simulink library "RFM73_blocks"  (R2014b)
settings: Solver=ode45  StartTime=0.0  StopTime=10.0  RelTol=1e-3
undefined symbols (not defined in the file): B, bin2dec, Model
libraries: simulink x5, RFM73_blocks x1, commutil2 x1, embdlinuxlib x1

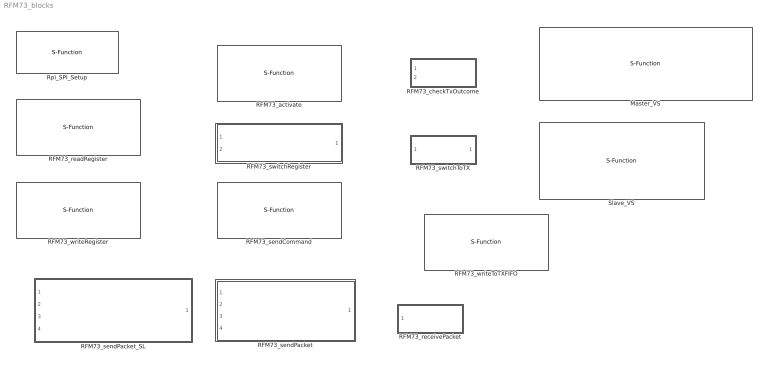
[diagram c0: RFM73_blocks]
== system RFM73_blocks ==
  Master_VS : S-Function  InitFcn=try, set_param(gcb,'FunctionName','RFM73_Master_VS'), end  FunctionName=RFM73_Master_VS  SFunctionModules=RFM73_Master_VS_wrapper  EnableBusSupport=off
  RFM73_activate : S-Function  InitFcn=try, set_param(gcb,'FunctionName','activate'), end  FunctionName=activate  SFunctionModules=activate_wrapper  EnableBusSupport=off
  RFM73_checkTxOutcome : Subsystem  TreatAsAtomicUnit=on
  RFM73_readRegister : S-Function  InitFcn=try, set_param(gcb,'FunctionName','readRegister'), end  FunctionName=readRegister  SFunctionModules=readRegister_wrapper  EnableBusSupport=off
  RFM73_receivePacket : Subsystem  TreatAsAtomicUnit=on
  RFM73_sendCommand : S-Function  InitFcn=try, set_param(gcb,'FunctionName','sendCommand'), end  FunctionName=sendCommand  SFunctionModules=sendCommand_wrapper  EnableBusSupport=off
  RFM73_sendPacket : Subsystem  TreatAsAtomicUnit=on
  RFM73_sendPacket_SL : Subsystem  TreatAsAtomicUnit=on
  RFM73_switchRegister : Subsystem
  RFM73_switchToTX : Subsystem  TreatAsAtomicUnit=on
  RFM73_writeRegister : S-Function  InitFcn=try, set_param(gcb,'FunctionName','writeRegister'), end  FunctionName=writeRegister  SFunctionModules=writeRegister_wrapper  EnableBusSupport=off
  RFM73_writeToTXFIFO : S-Function  InitFcn=try, set_param(gcb,'FunctionName','writeToTXFIFO'), end  FunctionName=writeToTXFIFO  SFunctionModules=writeToTXFIFO_wrapper  EnableBusSupport=off
  Rpi_SPI_Setup : S-Function  InitFcn=try, set_param(gcb,'FunctionName','SPI_interface_setup'), end  FunctionName=SPI_interface_setup  SFunctionModules=SPI_interface_setup_wrapper  EnableBusSupport=off
  Slave_VS : S-Function  InitFcn=try, set_param(gcb,'FunctionName','RFM73_Slave_VS'), end  FunctionName=RFM73_Slave_VS  SFunctionModules=RFM73_Slave_VS_wrapper  EnableBusSupport=off

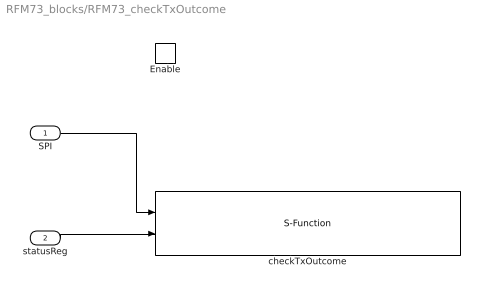
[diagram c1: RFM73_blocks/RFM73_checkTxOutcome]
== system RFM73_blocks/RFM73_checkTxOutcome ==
  SPI : Inport
  statusReg : Inport  Port=2
  Enable : EnablePort
  checkTxOutcome : S-Function  InitFcn=try, set_param(gcb,'FunctionName','checkTxOutcome'), end  FunctionName=checkTxOutcome  SFunctionModules=checkTxOutcome_wrapper  EnableBusSupport=off
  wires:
  SPI/1 -> checkTxOutcome/1
  statusReg/1 -> checkTxOutcome/2

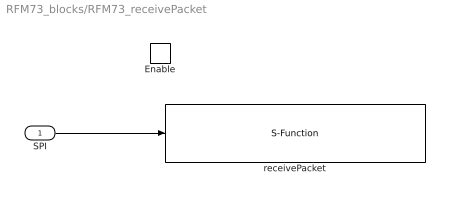
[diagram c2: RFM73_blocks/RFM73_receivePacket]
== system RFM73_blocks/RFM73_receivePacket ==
  SPI : Inport
  Enable : EnablePort
  receivePacket : S-Function  InitFcn=try, set_param(gcb,'FunctionName','receivePacket'), end  FunctionName=receivePacket  SFunctionModules=receivePacket_wrapper  EnableBusSupport=off
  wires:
  SPI/1 -> receivePacket/1

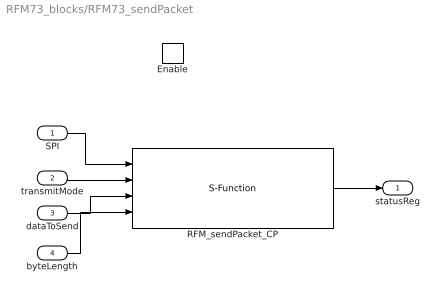
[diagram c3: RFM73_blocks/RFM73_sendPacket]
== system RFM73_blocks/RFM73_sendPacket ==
  SPI : Inport
  transmitMode : Inport  Port=2
  dataToSend : Inport  Port=3
  byteLength : Inport  Port=4
  Enable : EnablePort
  RFM_sendPacket_CP : S-Function  InitFcn=try, set_param(gcb,'FunctionName','sendPacket_CP'), end  FunctionName=sendPacket_CP  SFunctionModules=sendPacket_CP_wrapper  EnableBusSupport=off
  statusReg : Outport
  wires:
  RFM_sendPacket_CP/1 -> statusReg/1
  SPI/1 -> RFM_sendPacket_CP/1
  transmitMode/1 -> RFM_sendPacket_CP/2
  dataToSend/1 -> RFM_sendPacket_CP/3
  byteLength/1 -> RFM_sendPacket_CP/4

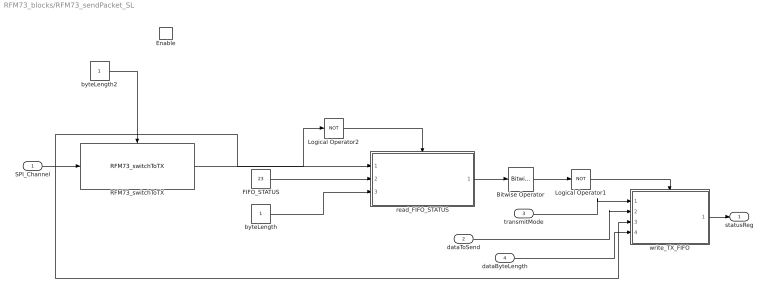
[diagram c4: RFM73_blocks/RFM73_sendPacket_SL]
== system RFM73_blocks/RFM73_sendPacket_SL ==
  SPI_Channel : Inport
  dataToSend : Inport  Port=2  OutDataTypeStr=uint8
  transmitMode : Inport  Port=3
  dataByteLength : Inport  Port=4  OutDataTypeStr=uint8
  Enable : EnablePort
  Bitwise Operator : simulink/Logic and Bit Operations/Bitwise Operator  logicop=AND  UseBitMask=on  BitMask=bin2dec('00000010')  BitMaskRealWorld=Stored Integer
  FIFO_STATUS : Constant  Value=23
  Logical Operator1 : Logic  Operator=NOT  AllPortsSameDT=off  OutDataTypeStr=boolean
  Logical Operator2 : Logic  Operator=NOT  AllPortsSameDT=off  OutDataTypeStr=boolean
  RFM73_switchToTX : RFM73_blocks/RFM73_switchToTX
      link override RFM73_sendCommand: FunctionName=sendCommand  SFunctionModules=sendCommand_wrapper
      link override RFM73_writeConfigRegister: FunctionName=writeRegister  SFunctionModules=writeRegister_wrapper
  byteLength : Constant
  byteLength2 : Constant
  read_FIFO_STATUS : Subsystem  TreatAsAtomicUnit=on
  write_TX_FIFO : Subsystem  TreatAsAtomicUnit=on
  statusReg : Outport
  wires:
  write_TX_FIFO/1(statusReg) -> statusReg/1
  dataByteLength/1 -> write_TX_FIFO/4(byteLength)
  transmitMode/1 -> write_TX_FIFO/1(type)
  dataToSend/1 -> write_TX_FIFO/2(data)
  Logical Operator1/1 -> write_TX_FIFO/Enable
  Bitwise Operator/1 -> Logical Operator1/1
  read_FIFO_STATUS/1(regContent) -> Bitwise Operator/1
  Logical Operator2/1 -> read_FIFO_STATUS/Enable
  RFM73_switchToTX/1 -> Logical Operator2/1
  byteLength/1 -> read_FIFO_STATUS/3(byteLength)
  FIFO_STATUS/1 -> read_FIFO_STATUS/2(regAddress)
  SPI_Channel/1 -> RFM73_switchToTX/1, read_FIFO_STATUS/1(SPI_Channel), write_TX_FIFO/3(SPI_Channel)
  byteLength2/1 -> RFM73_switchToTX/Enable

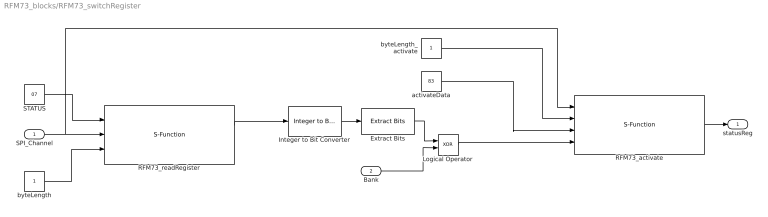
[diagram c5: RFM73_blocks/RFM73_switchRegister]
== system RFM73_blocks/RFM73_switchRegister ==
  SPI_Channel : Inport
  Bank : Inport  Port=2
  Extract Bits : simulink/Logic and Bit Operations/Extract Bits  bitsToExtract=Range of bits  numBits=8  bitIdxRange=[7]  outScalingMode=Preserve fixed-point scaling
  Integer to Bit Converter : commutil2/Integer to Bit Converter  nbits=8  signedInputValues=Unsigned  bitOrder=MSB first  outDtype=Inherit via internal rule
  Logical Operator : Logic  Operator=XOR  IconShape=distinctive  AllPortsSameDT=off  OutDataTypeStr=boolean
  RFM73_activate : S-Function  InitFcn=try, set_param(gcb,'FunctionName','activate'), end  FunctionName=activate  SFunctionModules=activate_wrapper  EnableBusSupport=off
  RFM73_readRegister : S-Function  InitFcn=try, set_param(gcb,'FunctionName','readRegister'), end  FunctionName=readRegister  SFunctionModules=readRegister_wrapper  EnableBusSupport=off
  STATUS : Constant  Value=07
  activateData : Constant  Value=83
  byteLength : Constant
  byteLength_activate : Constant
  statusReg : Outport
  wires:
  SPI_Channel/1 -> RFM73_activate/1, RFM73_readRegister/2
  STATUS/1 -> RFM73_readRegister/1
  byteLength/1 -> RFM73_readRegister/3
  RFM73_readRegister/1 -> Integer to Bit Converter/1
  Integer to Bit Converter/1 -> Extract Bits/1
  Extract Bits/1 -> Logical Operator/1
  Bank/1 -> Logical Operator/2
  byteLength_activate/1 -> RFM73_activate/2
  activateData/1 -> RFM73_activate/3
  Logical Operator/1 -> RFM73_activate/4
  RFM73_activate/1 -> statusReg/1

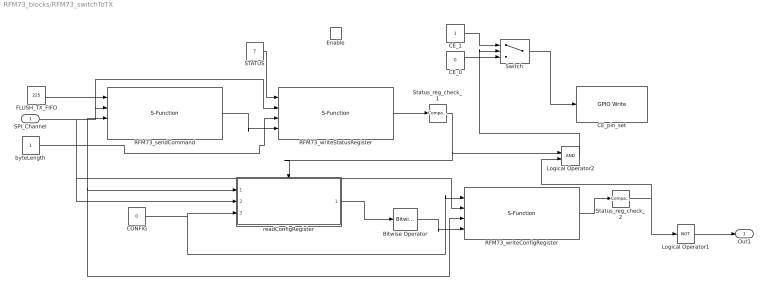
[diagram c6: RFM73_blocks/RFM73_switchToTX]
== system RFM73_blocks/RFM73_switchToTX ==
  SPI_Channel : Inport
  Enable : EnablePort
  Bitwise Operator : simulink/Logic and Bit Operations/Bitwise Operator  logicop=AND  UseBitMask=on  BitMask=bin2dec('11111110')  BitMaskRealWorld=Stored Integer
  CE_0 : Constant  Value=0  OutDataTypeStr=boolean
  CE_1 : Constant  OutDataTypeStr=boolean
  CE_pin_set : embdlinuxlib/GPIO Write  board=Model B+  gpio=23  direction=Output  blockPlatform=Raspberry Pi
  CONFIG : Constant  Value=0
  FLUSH_TX_FIFO : Constant  Value=225
  Logical Operator1 : Logic  Operator=NOT  AllPortsSameDT=off  OutDataTypeStr=boolean
  Logical Operator2 : Logic  AllPortsSameDT=off  OutDataTypeStr=fixdt(0,16)
  RFM73_sendCommand : S-Function  InitFcn=try, set_param(gcb,'FunctionName','sendCommand'), end  FunctionName=sendCommand  SFunctionModules=sendCommand_wrapper  EnableBusSupport=off
  RFM73_writeConfigRegister : S-Function  InitFcn=try, set_param(gcb,'FunctionName','writeRegister'), end  FunctionName=writeRegister  SFunctionModules=writeRegister_wrapper  EnableBusSupport=off
  RFM73_writeStatusRegister : S-Function  InitFcn=try, set_param(gcb,'FunctionName','writeRegister'), end  FunctionName=writeRegister  SFunctionModules=writeRegister_wrapper  EnableBusSupport=off
  STATUS : Constant  Value=7
  Status_reg_check_1 : simulink/Logic and Bit Operations/Compare To Constant  relop===  const=14  OutDataTypeStr=uint8
  Status_reg_check_2 : simulink/Logic and Bit Operations/Compare To Constant  relop===  const=14  OutDataTypeStr=uint8
  Switch : Switch  Criteria=u2 ~= 0
  byteLength : Constant
  readConfigRegister : Subsystem  TreatAsAtomicUnit=on
  Out1 : Outport
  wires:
  SPI_Channel/1 -> RFM73_writeConfigRegister/2, readConfigRegister/2(SPI_Channel), RFM73_writeStatusRegister/2, RFM73_sendCommand/2
  FLUSH_TX_FIFO/1 -> RFM73_sendCommand/1
  byteLength/1 -> RFM73_writeConfigRegister/3, readConfigRegister/1(byteLength), RFM73_writeStatusRegister/3, RFM73_sendCommand/3
  STATUS/1 -> RFM73_writeStatusRegister/1
  RFM73_sendCommand/1 -> RFM73_writeStatusRegister/4
  RFM73_writeStatusRegister/1 -> Status_reg_check_1/1
  Status_reg_check_1/1 -> readConfigRegister/Enable, Logical Operator2/1
  CONFIG/1 -> RFM73_writeConfigRegister/1, readConfigRegister/3(regAddress)
  readConfigRegister/1(regContent) -> Bitwise Operator/1
  Bitwise Operator/1 -> RFM73_writeConfigRegister/4
  RFM73_writeConfigRegister/1 -> Status_reg_check_2/1
  Status_reg_check_2/1 -> Logical Operator2/2, Logical Operator1/1
  Logical Operator1/1 -> Out1/1
  CE_0/1 -> Switch/3
  CE_1/1 -> Switch/1
  Switch/1 -> CE_pin_set/1
  Logical Operator2/1 -> Switch/2

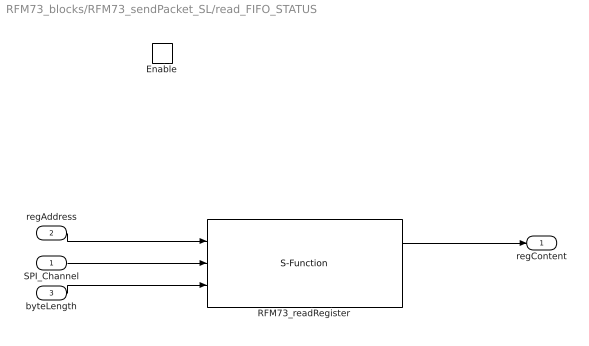
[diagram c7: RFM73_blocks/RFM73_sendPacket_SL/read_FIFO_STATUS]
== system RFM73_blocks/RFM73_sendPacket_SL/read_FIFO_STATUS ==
  SPI_Channel : Inport
  regAddress : Inport  Port=2
  byteLength : Inport  Port=3
  Enable : EnablePort
  RFM73_readRegister : S-Function  InitFcn=try, set_param(gcb,'FunctionName','readRegister'), end  FunctionName=readRegister  SFunctionModules=readRegister_wrapper  EnableBusSupport=off
  regContent : Outport
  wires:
  byteLength/1 -> RFM73_readRegister/3
  regAddress/1 -> RFM73_readRegister/1
  SPI_Channel/1 -> RFM73_readRegister/2
  RFM73_readRegister/1 -> regContent/1

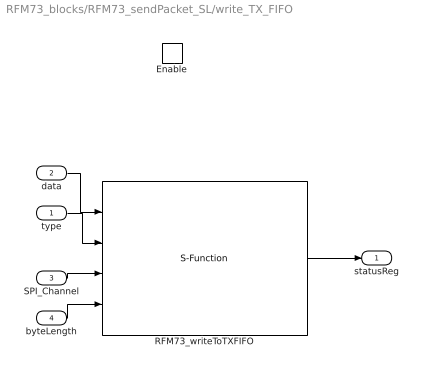
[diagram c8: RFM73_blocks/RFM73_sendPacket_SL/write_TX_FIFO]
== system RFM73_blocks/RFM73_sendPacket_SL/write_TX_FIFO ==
  type : Inport
  data : Inport  Port=2  OutDataTypeStr=uint8
  SPI_Channel : Inport  Port=3
  byteLength : Inport  Port=4  OutDataTypeStr=uint8
  Enable : EnablePort
  RFM73_writeToTXFIFO : S-Function  InitFcn=try, set_param(gcb,'FunctionName','writeToTXFIFO'), end  FunctionName=writeToTXFIFO  SFunctionModules=writeToTXFIFO_wrapper  EnableBusSupport=off
  statusReg : Outport
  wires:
  RFM73_writeToTXFIFO/1 -> statusReg/1
  byteLength/1 -> RFM73_writeToTXFIFO/4
  SPI_Channel/1 -> RFM73_writeToTXFIFO/3
  data/1 -> RFM73_writeToTXFIFO/1
  type/1 -> RFM73_writeToTXFIFO/2

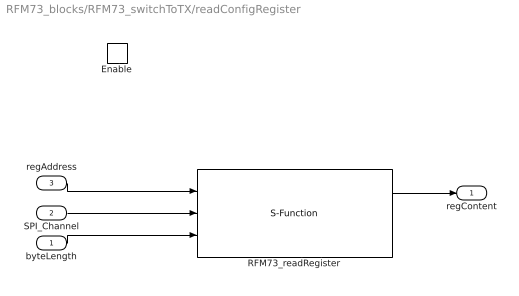
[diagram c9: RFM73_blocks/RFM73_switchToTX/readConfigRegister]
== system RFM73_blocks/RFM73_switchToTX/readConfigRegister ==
  byteLength : Inport
  SPI_Channel : Inport  Port=2
  regAddress : Inport  Port=3
  Enable : EnablePort
  RFM73_readRegister : S-Function  InitFcn=try, set_param(gcb,'FunctionName','readRegister'), end  FunctionName=readRegister  SFunctionModules=readRegister_wrapper  EnableBusSupport=off
  regContent : Outport
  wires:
  byteLength/1 -> RFM73_readRegister/3
  SPI_Channel/1 -> RFM73_readRegister/2
  regAddress/1 -> RFM73_readRegister/1
  RFM73_readRegister/1 -> regContent/1
